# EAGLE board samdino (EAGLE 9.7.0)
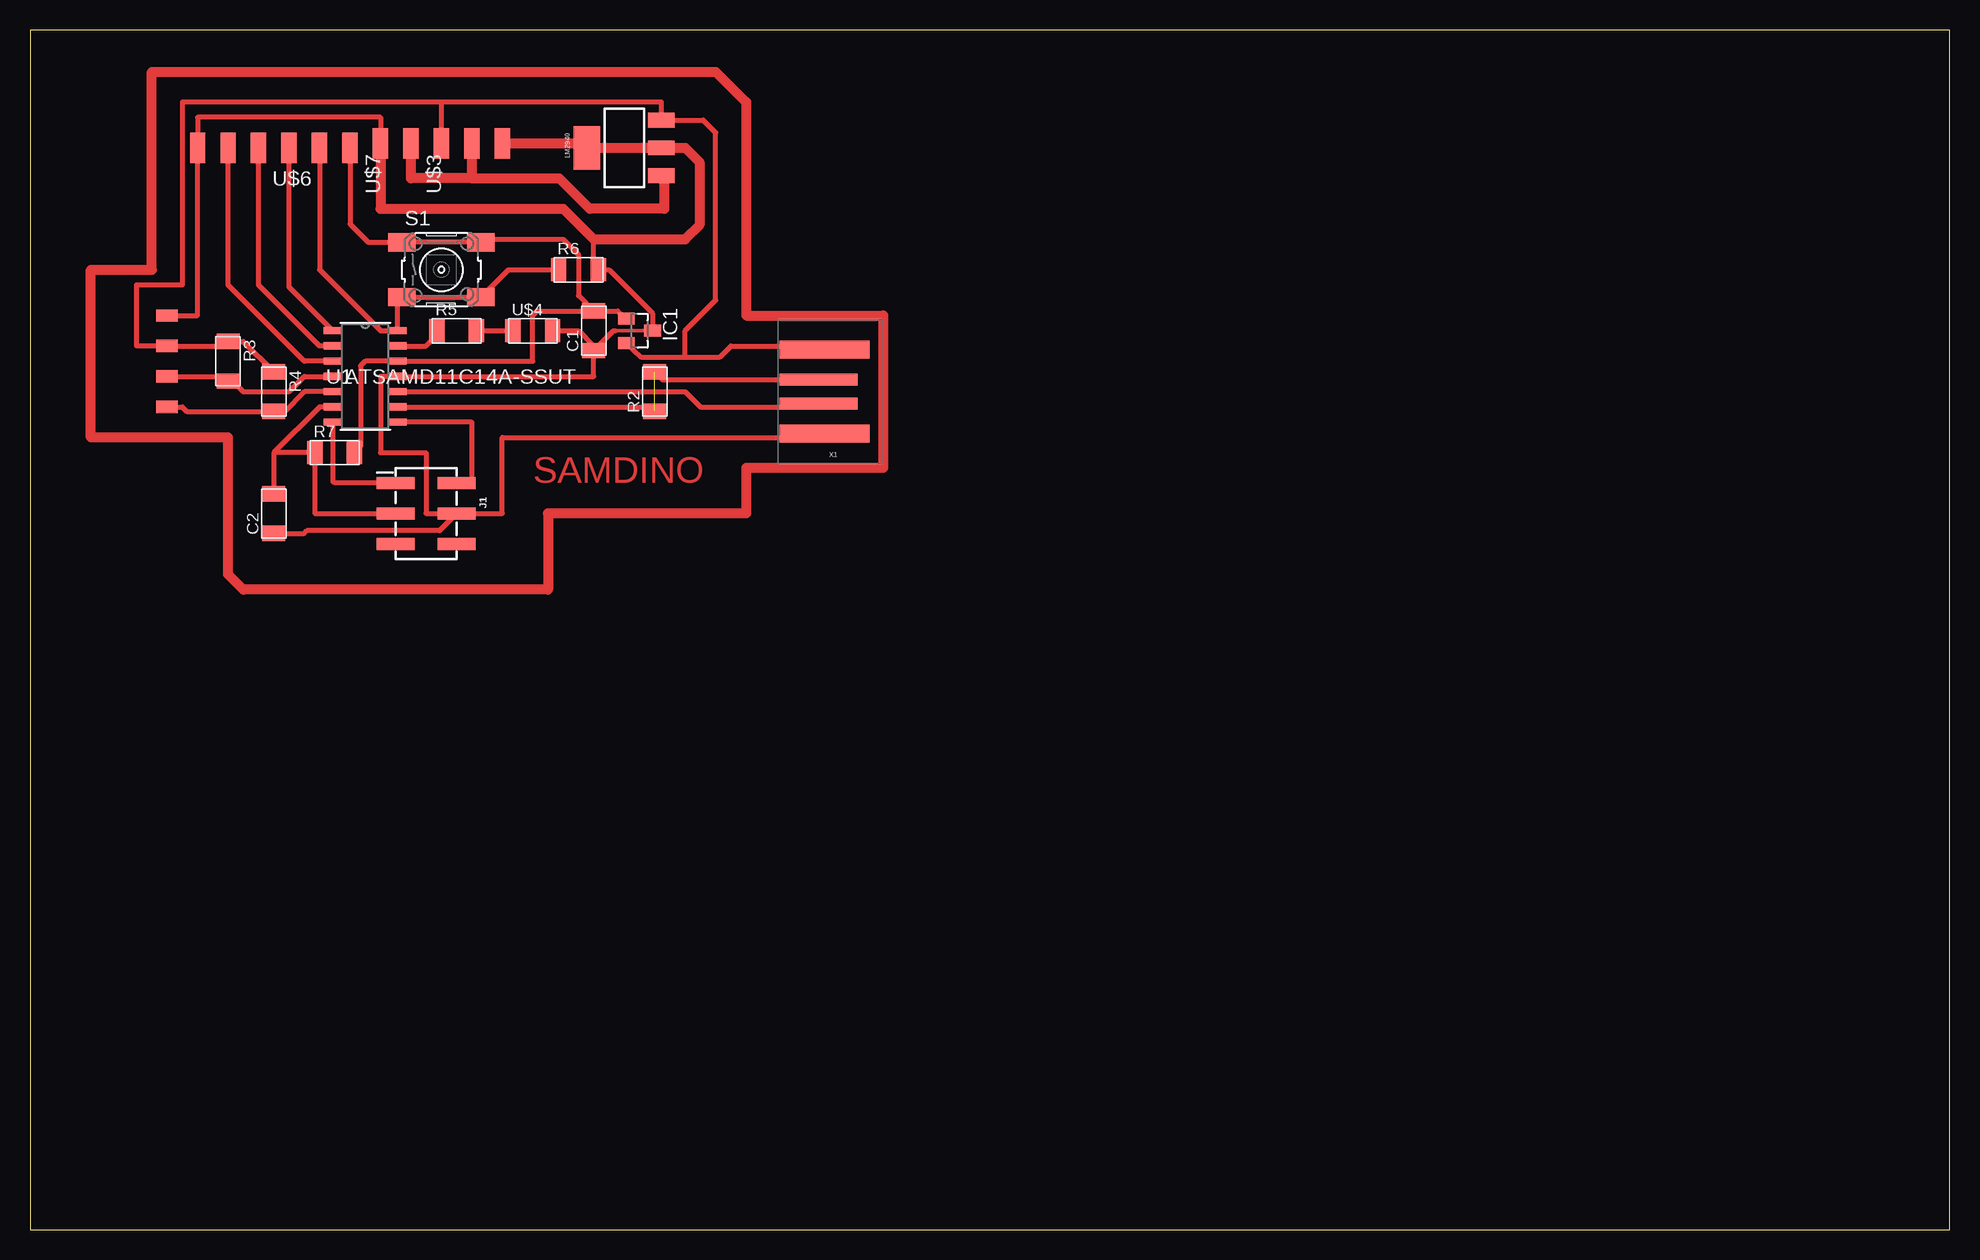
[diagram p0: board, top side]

Size 160 x 100 mm. Coordinates in mm from the lower left corner, seen from the top.
Outline: 0,0 160,0 160,100 0,100 0,0
Copper layers (1*16): Top / Bottom
Stack-up Default Layer Stack: Top User Defined 0.035mm / Dielectric-1 User Defined 1.5mm / Bottom User Defined 0.035mm
Design rules: minimum copper width 16mil, minimum drill size 0.35mm, copper clearance wire_polygon to wire_polygon 16mil, copper clearance wire_polygon to pad_smd 16mil, copper clearance wire_polygon to via 16mil, copper clearance pad_smd to pad_smd 16mil, copper clearance pad_smd to via 16mil, copper clearance via to via 16mil, copper clearance smd to pad (same net) 6mil, copper clearance smd to via (same net) 6mil, copper clearance smd to smd (same net) 6mil, dimension clearance 40mil, restrict clearance 0mil, drill distance 16mil, keepout clearance 0mil

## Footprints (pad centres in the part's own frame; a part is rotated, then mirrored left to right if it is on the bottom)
C1206FAB = smd 1.27 x 1.905: 1 -1.651,0; 2 1.651,0
SOT23 = smd 1 x 1.4: 1 -1.001,-1.1; 2 1.014,-1.1; 3 0,1.1
2X3_SMT_POSTS = smd 1 x 3.17: 1 -2.54,-2.54; 2 -2.54,2.54; 3 0,-2.54; 4 0,2.54; 5 2.54,-2.54; 6 2.54,2.54
1X04SMD/90 = smd 1.016 x 1.778: 1 -1.27,-5.08; 2 1.27,-5.08; 3 3.81,-5.08; 4 6.35,-5.08
SOT223 = smd 1.219 x 2.235: 1 -2.311,-3.099; 2 0,-3.099; 3 2.311,-3.099 | smd 3.6 x 2.2: 4 0,3.099
R1206FAB = smd 1.27 x 1.905: 1 -1.651,0; 2 1.651,0
6MM_SWITCH = smd 2.286 x 1.524: 1 -3.302,2.286; 2 3.302,2.286; 3 -3.302,-2.286; 4 3.302,-2.286
SOIC14_SL_MCH = smd 1.5 x 0.6: 1 -2.7,3.81; 2 -2.7,2.54; 3 -2.7,1.27; 4 -2.7,0; 5 -2.7,-1.27; 6 -2.7,-2.54; 7 -2.7,-3.81; 8 2.7,-3.81; 9 2.7,-2.54; 10 2.7,-1.27; 11 2.7,0; 12 2.7,1.27; 13 2.7,2.54; 14 2.7,3.81
SPDTSWITCH = smd 2.54 x 1.27: 1 0.38,2.54; 2 0.38,0; 3 0.38,-2.54
LED1206FAB = smd 1.27 x 1.905: 1 -1.651,0; 2 1.651,0
1X06SMD = smd 2.54 x 1.27: 1 0,6.35; 2 0,3.81; 3 0,1.27; 4 0,-1.27; 5 0,-3.81; 6 0,-6.35
USB-A-PCB = smd 7.5 x 1.5: 5V -0.2,-3.5; GND -0.2,3.5 | smd 6.5 x 1: USB_M 0.3,-1; USB_P 0.3,1

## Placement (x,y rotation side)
C1  1uF  [C1206FAB]  46.99,74.93 90 top
C2  1uF  [C1206FAB]  20.32,59.69 90 top
IC1  [SOT23]  50.8,74.93 270 top
J1  [2X3_SMT_POSTS]  33.02,59.69 270 top
JP3  [1X04SMD/90]  16.51,74.93 270 top
LM2940  VR_REGULATOR_SOT223  [SOT223]  49.53,90.17 90 top
R2  0  [R1206FAB]  52.07,69.85 90 top
R3  4.99K  [R1206FAB]  16.51,72.39 270 top
R4  4.99K  [R1206FAB]  20.32,69.85 270 top
R5  1K  [R1206FAB]  35.56,74.93 0 top
R6  470  [R1206FAB]  45.72,80.01 0 top
R7  10K  [R1206FAB]  25.4,64.77 0 top
S1  [6MM_SWITCH]  34.29,80.01 0 top
U1  ATSAMD11C14A-SSUT  [SOIC14_SL_MCH]  27.94,71.12 0 top
U$3  SPDTSWITCH  [SPDTSWITCH]  36.83,90.17 90 top
U$4  LEDFAB1206  [LED1206FAB]  41.91,74.93 0 top
U$6  CONN_06_FTDI-SMD-HEADER  [1X06SMD]  20.32,90.17 90 top
U$7  SPDTSWITCH  [SPDTSWITCH]  31.75,90.17 90 top
X1  CONN_USBPCB  [USB-A-PCB]  66.04,69.85 180 top

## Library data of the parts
C1 C2 IC1 LM2940 R2-R7 S1 U$3 U$4 U$6 U$7 X1 = fab
J1 = fab; PROD_ID: CONN-11415
JP3 = pinhead-2
U1 = samd11c; BUILT_BY: EMA_Molly; COPYRIGHT: Copyright (C) 2018 Accelerated Designs. All rights reserved; MANUFACTURER_PART_NUMBER: ATSAMD11C14A-SSUT; SOURCELIBRARY: Microchip_2019-08-23_25; VENDOR: Microchip

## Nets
2: R5.1 U1.13
4: R6.1 S1.3 S1.4 U1.14 U$6.5
5: U1.1 U$6.4
5V: IC1.2 JP3.2 LM2940.3 R3.1 R4.1 U$3.1 U$7.3 X1.5V
8: U1.2 U$6.3
9: U1.3 U$6.2
24-: R2.1 R2.2 U1.9 X1.USB_M
25+: U1.10 X1.USB_P
CLK: J1.1 U1.7
DIO: J1.2 U1.8
GND: C1.1 C2.1 IC1.3 J1.4 JP3.1 LM2940.2 LM2940.4 R6.2 U1.11 U$3.3 U$4.2 U$6.1 U$7.1 X1.GND
N$5: R5.2 U$4.1
RST: C2.2 J1.3 R7.1 U1.6
SCL: JP3.4 R4.2 U1.5
SDA: JP3.3 R3.2 U1.4
VD0: LM2940.1 U$3.2 U$7.2
VDD: C1.2 IC1.1 R7.2 S1.1 S1.2 U1.12 U$6.6

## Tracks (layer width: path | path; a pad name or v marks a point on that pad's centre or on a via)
2
  Top 0.406: U1.13 33.02,73.66 33.91,74.55 R5.1
4
  Top 0.406: S1.3 30.64,77.38 U1.14 29.21,74.93 24.13,80.01 U$6.5 | S1.3 31.24,77.47 | S1.3 31.5,77.72 | S1.3 S1.4 39.88,80.01 R6.1
5
  Top 0.406: U1.1 21.59,78.58 U$6.4
5V
  Top 0.406: X1.5V 65.93,73.66 58.42,73.66 57.51,72.75 54.61,72.75 | IC1.2 50.93,72.75 54.61,72.75 | 54.61,72.75 54.61,74.93 57.15,77.47 57.15,91.44 56.11,92.48 LM2940.3 52.63,93.98 34.29,93.98 | 34.29,93.98 U$7.3 | R4.1 17.78,74.04 R3.1 16.13,73.66 JP3.2 8.89,73.66 8.89,78.74 12.7,78.74 12.7,93.98 34.29,93.98
8
  Top 0.406: U1.2 24.13,73.66 19.05,78.74 U$6.3
9
  Top 0.406: U1.3 22.86,72.39 16.51,78.74 U$6.2
24-  (1 unrouted)
  Top 0.406: 30.48,68.58 U1.9 51.69,68.58 R2.1 | R2.2 52.72,70.85 X1.USB_M
25+
  Top 0.406: U1.10 54.61,69.85 55.88,68.58 65.47,68.58 X1.USB_P
CLK
  Top 0.406: 25.24,67.15 U1.7 25.24,62.39 25.4,62.23 J1.1
DIO
  Top 0.406: U1.8 36.83,67.31 36.83,62.23 J1.2
GND
  Top 0.305: 48.79,74.92 IC1.3
  Top 0.406: X1.GND 65.93,66.04 39.37,66.04 39.37,59.69 J1.4 | C1.1 46.99,71.12 U1.11 29.21,71.12 29.21,64.77 33.02,64.77 33.02,59.69 J1.4 | C1.1 46.99,73.66 45.72,74.93 U$4.2 | C1.1 48.63,74.92 48.79,74.92 | 52.07,75.1 IC1.3 51.89,76.38 48.26,80.01 R6.2 46.99,80.39 46.99,82.55 | U$7.1 29.21,92.71 13.97,92.71 U$6.1 13.97,76.2 JP3.1 | C2.1 22.86,58.04 23.08,58.26 34.13,58.26 J1.4
  Top 0.813: U$3.3 46.43,90.55 LM2940.4 LM2940.2 54.61,90.17 55.8,88.98 55.8,83.74 54.61,82.55 46.99,82.55 44.45,85.09 29.21,85.09 U$7.1
N$1
  Top 0.813: 10.16,96.52 57.15,96.52 59.69,93.98 59.69,76.2 71.12,76.2 71.12,63.5 59.69,63.5 59.69,59.69 43.18,59.69 43.18,53.34 17.78,53.34 16.51,54.61 16.51,66.04 5.08,66.04 5.08,80.01 10.16,80.01 10.16,96.52
N$5
  Top 0.406: R5.2 U$4.1
RST
  Top 0.406: U1.6 24.13,68.58 20.32,64.77 | 20.32,64.77 C2.2 | 20.32,64.77 R7.1 23.75,59.69 J1.3
SCL
  Top 0.406: U1.5 22.86,69.85 21.21,68.2 R4.2 13.08,68.2 12.7,68.58 JP3.4
SDA
  Top 0.406: U1.4 22.86,71.12 21.59,69.85 17.78,69.85 16.89,70.74 R3.2 16.13,71.12 JP3.3
VD0
  Top 0.813: U$3.2 36.83,87.63 | 36.83,87.63 44.12,87.63 46.66,85.09 52.86,85.09 52.86,87.63 LM2940.1 | 36.83,87.63 31.75,87.63 U$7.2
VDD
  Top 0.406: 49.38,76.2 IC1.1 49,76.58 C1.2 | C1.2 42.29,76.58 41.91,76.2 41.91,72.39 U1.12 27.94,72.39 27.56,72.01 27.56,65.28 R7.2 | C1.2 45.72,77.85 45.72,81.28 44.45,82.55 37.85,82.55 S1.2 S1.1 28.19,82.3 26.67,83.82 U$6.6

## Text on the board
Top: SAMDINO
